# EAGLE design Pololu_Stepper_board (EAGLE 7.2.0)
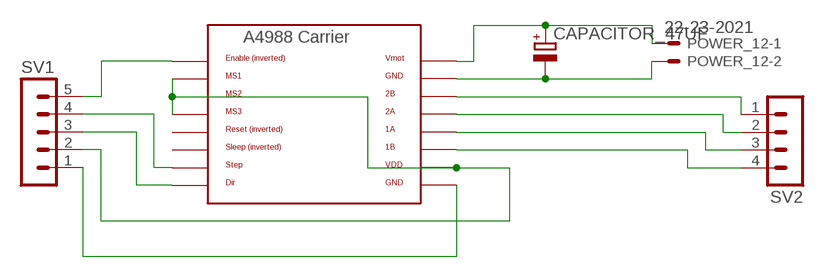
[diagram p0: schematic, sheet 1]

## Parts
CAPACITOR_47UF  CPOL-EUB  [PANASONIC_B]
POWER_12  22-23-2021  [22-23-2021]
SV1  MA05-1  [MA05-1]
SV2  MA04-1  [MA04-1]
XAXIS  A4988BREAKOUT  [A4988BREAKOUT]

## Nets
MOTOR_POLOLU: SV2.1 XAXIS.2B
N$1: CAPACITOR_47UF.+ POWER_12.1 XAXIS.VMOT
N$2: CAPACITOR_47UF.- POWER_12.2 XAXIS.GND@0(GND)
N$4: SV2.2 XAXIS.2A
N$5: SV2.3 XAXIS.1A
N$6: SV2.4 XAXIS.1B
N$7: SV1.5 XAXIS.EN
N$8: SV1.4 XAXIS.STEP
N$9: SV1.3 XAXIS.DIR
SASCHAKIT: SV1.1 XAXIS.GND
VCC: SV1.2 XAXIS.MS1 XAXIS.MS2 XAXIS.MS3 XAXIS.VDD
Unconnected: XAXIS.RST XAXIS.SLP(SLEEP)

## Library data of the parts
CAPACITOR_47UF = rcl:CPOL-EU: POLARIZED CAPACITOR, European symbol
POWER_12 = con-molex:22-23-2021: .100" (2.54mm) Center Header - 2 Pin; MF: MOLEX; MPN: 22-23-2021; OC_FARNELL: 1462926; OC_NEWARK: 25C3832
SV1 = con-lstb:MA05-1: PIN HEADER; OC_FARNELL: unknown; OC_NEWARK: unknown
SV2 = con-lstb:MA04-1: PIN HEADER; OC_FARNELL: unknown; OC_NEWARK: unknown
XAXIS = RepRapjr:A4988BREAKOUT

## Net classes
0 default: width 0.254 mm, drill 0.254 mm, clearance 0.254 mm
1 power: width 0.254 mm, drill 0.254 mm, clearance 0.254 mm
2 gnd: width 0.254 mm, drill 0.254 mm, clearance 0.254 mm
3 usbvcc: width 0.254 mm, drill 0.254 mm, clearance 0.254 mm
4 aref: width 0.254 mm, drill 0.254 mm, clearance 0.254 mm

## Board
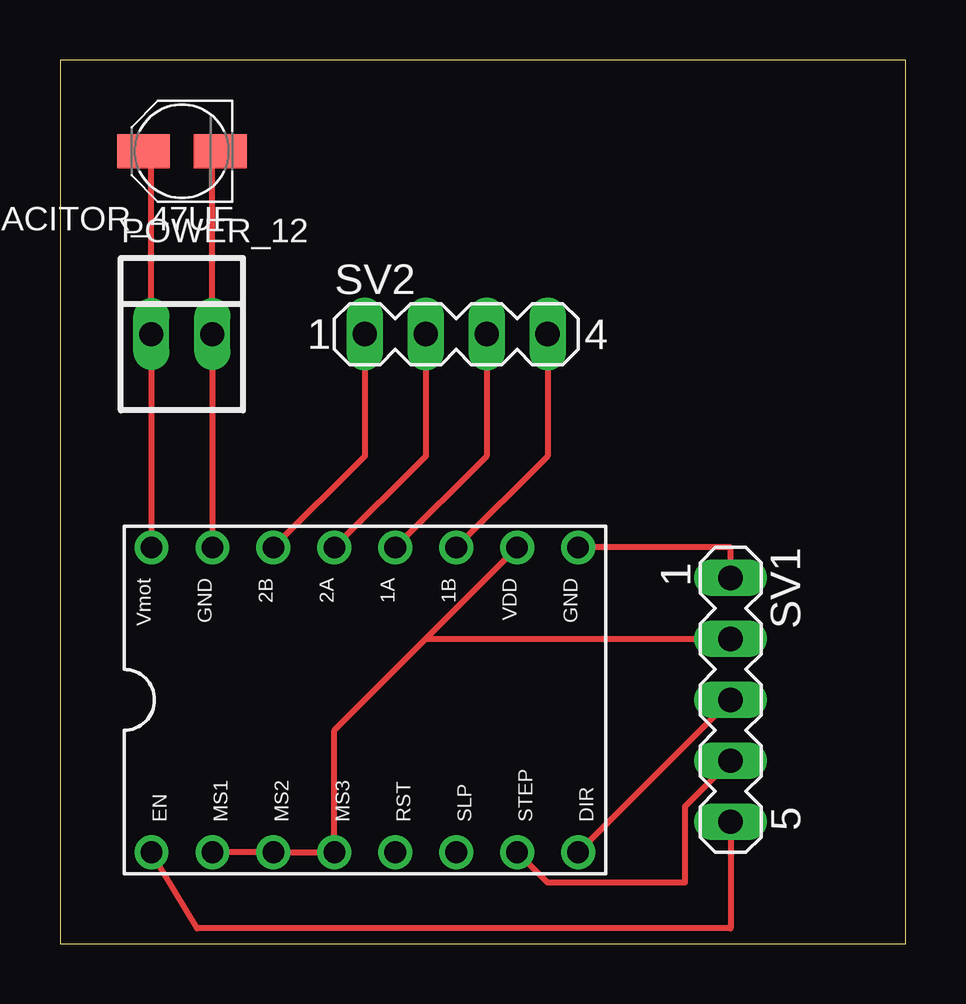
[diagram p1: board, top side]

Size 35.23 x 36.82 mm. Coordinates in mm from the lower left corner, seen from the top.
Outline: 0,0 35.23,0 35.23,36.82 0,36.82 0,0
Copper layers (1*16): Top 0.035mm / dielectric 1.5mm / Bottom 0.035mm
Design rules "default": minimum track width 10mil, minimum drill 24mil, track to track 8mil, track to pad 8mil, pad to pad 8mil, via to via 8mil, smd to smd 8mil, copper to edge 40mil, drill to drill 8mil, minimum pad ring 10mil, minimum via ring 8mil, stop-mask expansion 4mil, vias tented up to drill 0mil, thermal gap 10mil

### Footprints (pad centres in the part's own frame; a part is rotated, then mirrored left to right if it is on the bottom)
PANASONIC_B = smd 2.2 x 1.4: + 1.6,0; - -1.6,0
22-23-2021 = drill 1 long: 1 -1.27,0; 2 1.27,0
MA05-1 = drill 1.016 long: 1 -5.08,0; 2 -2.54,0; 3 0,0; 4 2.54,0; 5 5.08,0
MA04-1 = drill 1.016 long: 1 -3.81,0; 2 -1.27,0; 3 1.27,0; 4 3.81,0
A4988BREAKOUT = drill 0.9: 1A 8.89,1.27; 1B 11.43,1.27; 2A 6.35,1.27; 2B 3.81,1.27; DIR 16.51,-11.43; EN -1.27,-11.43; GND 16.51,1.27; GND@0 1.27,1.27; MS1 1.27,-11.43; MS2 3.81,-11.43; MS3 6.35,-11.43; RST 8.89,-11.43; SLP 11.43,-11.43; STEP 13.97,-11.43; VDD 13.97,1.27; VMOT -1.27,1.27

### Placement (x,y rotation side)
CAPACITOR_47UF  5.08,33.02 180 top
POWER_12  5.08,25.4 0 top
SV1  27.94,10.16 270 top
SV2  16.51,25.4 0 top
XAXIS  5.08,15.24 0 top

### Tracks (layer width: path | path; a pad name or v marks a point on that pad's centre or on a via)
MOTOR_POLOLU
  Top 0.254: XAXIS.2B 12.7,20.32 SV2.1
N$1
  Top 0.254: CAPACITOR_47UF.+ 3.81,33.02 POWER_12.1 XAXIS.VMOT
N$2
  Top 0.254: CAPACITOR_47UF.- 6.35,33.02 POWER_12.2 XAXIS.GND@0
N$4
  Top 0.254: XAXIS.2A 15.24,20.32 SV2.2
N$5
  Top 0.254: XAXIS.1A 17.78,20.32 SV2.3
N$6
  Top 0.254: SV2.4 20.32,20.32 XAXIS.1B
N$7
  Top 0.254: XAXIS.EN 5.72,0.63 27.94,0.63 SV1.5
N$8
  Top 0.254: XAXIS.STEP 20.32,2.54 26.03,2.54 26.03,5.71 SV1.4
N$9
  Top 0.254: SV1.3 XAXIS.DIR
SASCHAKIT
  Top 0.254: XAXIS.GND 27.94,16.51 SV1.1
VCC
  Top 0.254: XAXIS.MS1 XAXIS.MS2 XAXIS.MS3 11.43,8.89 15.24,12.7 | 15.24,12.7 XAXIS.VDD | 15.24,12.7 SV1.2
